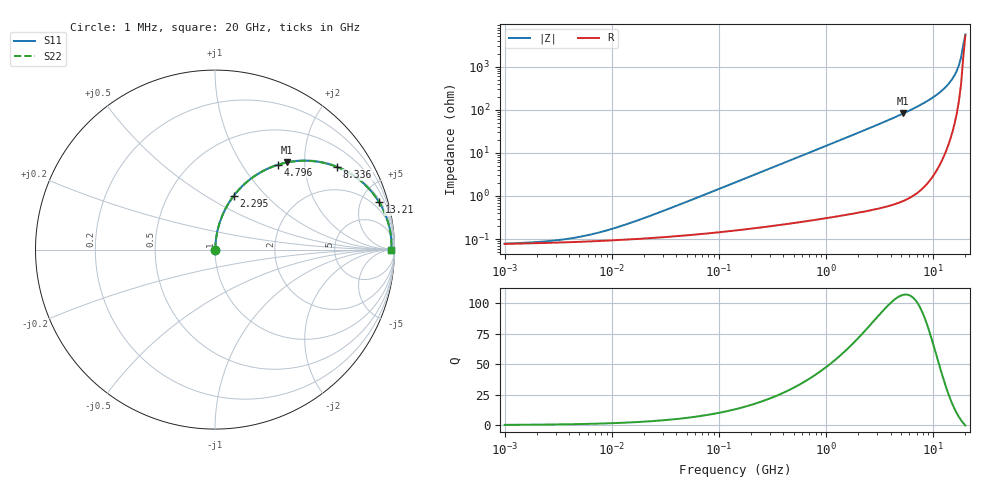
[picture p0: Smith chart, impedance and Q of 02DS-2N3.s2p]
# MHz S MA R 50
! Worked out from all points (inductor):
!   216 points, 1 MHz to 20 GHz, reference 50 ohm
!   read as one part in series: L = 2.3 nH near 21.89 MHz
!   highest Q = 107 at 5.259 GHz (marker M1), where L = 2.47 nH
!   self-resonance near 19.1 GHz
!   S11 on the Smith chart (normalised r, x): 1 MHz: 1.00, +0.00; 2.295 GHz: 1.01, +0.67; 4.796 GHz: 1.01, +1.47; 8.336 GHz: 1.03, +2.93; 13.21 GHz: 1.22, +6.85; 20 GHz: open
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1  0.0007868 10.6  0.9992 -0.0  0.9992 -0.0  0.0007868 10.6
2.51244  0.0008936 23.9  0.9992 -0.0  0.9992 -0.0  0.0008936 23.9
5.25016  0.001153 41.1  0.9991 -0.0  0.9991 -0.0  0.001153 41.1
10.9711  0.001844 59.1  0.9991 -0.1  0.9991 -0.1  0.001844 59.1
27.5642  0.004125 74.5  0.9989 -0.2  0.9989 -0.2  0.004125 74.5
144.716  0.02094 84.5  0.9982 -1.2  0.9982 -1.2  0.02094 84.5
759.783  0.109 82.3  0.9913 -6.3  0.9913 -6.3  0.109 82.3
1447.96  0.2052 77.2  0.9753 -11.8  0.9753 -11.8  0.2052 77.2
2295.12  0.3174 70.7  0.9442 -18.5  0.9442 -18.5  0.3174 70.7
3988.98  0.5127 58.6  0.8534 -30.8  0.8534 -30.8  0.5127 58.6
4796.03  0.5902 53.3  0.8017 -36.2  0.8017 -36.2  0.5902 53.3
5258.85  0.63 50.4  0.7707 -39.0  0.7707 -39.0  0.63 50.4
6620.87  0.7293 42.6  0.6773 -46.8  0.6773 -46.8  0.7293 42.6
8335.64  0.8212 34.1  0.5614 -55.2  0.5614 -55.2  0.8212 34.1
10989.2  0.9103 23.4  0.3974 -65.5  0.3974 -65.5  0.9103 23.4
13212.6  0.9518 16.1  0.2776 -72.0  0.2776 -72.0  0.9518 16.1
14487.6  0.9664 12.4  0.2158 -74.9  0.2158 -74.9  0.9664 12.4
15885.7  0.9766 8.8  0.1533 -76.9  0.1533 -76.9  0.9766 8.8
17418.7  0.9825 5.1  0.0907 -76.3  0.0907 -76.3  0.9825 5.1
18239.8  0.9837 3.3  0.05988 -72.6  0.05988 -72.6  0.9837 3.3
19099.6  0.9839 1.5  0.0308 -57.8  0.0308 -57.8  0.9839 1.5
20000  0.983 -0.3  0.01775 16.2  0.01775 16.2  0.983 -0.3
